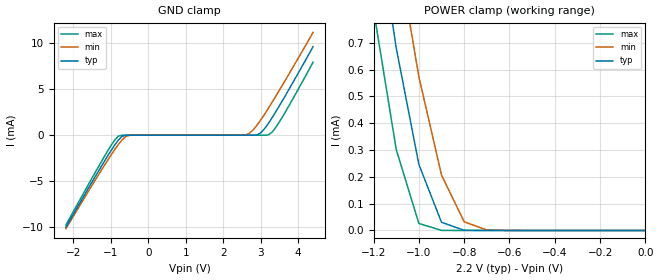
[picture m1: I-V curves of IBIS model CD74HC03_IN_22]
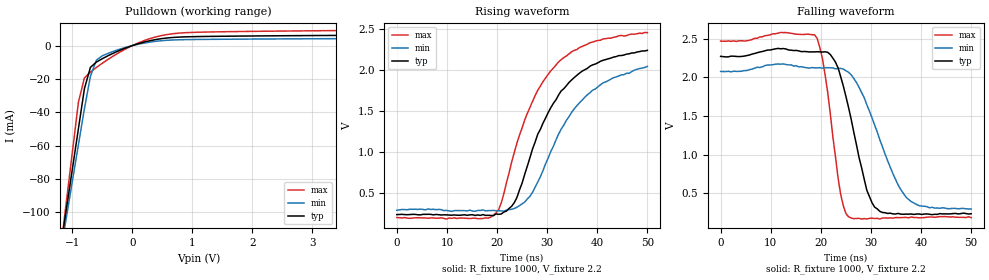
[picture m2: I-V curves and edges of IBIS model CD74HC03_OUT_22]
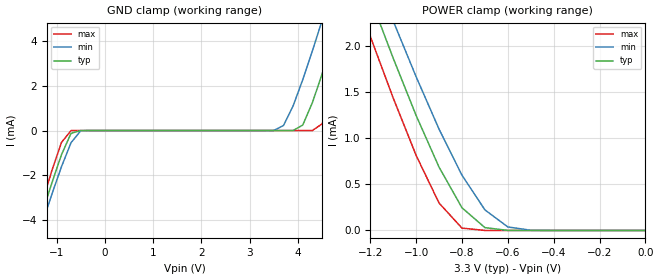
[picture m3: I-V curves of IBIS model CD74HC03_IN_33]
|   TEXAS INSTRUMENTS INCORPORATED
|   Standard Linear and Logic
|   IBIS Model of CD74HC03
|   HIGH SPEED CMOS LOGIC
|   QUAD 2-INPUT NAND GATE WITH OPEN DRAIN
|   DIP 14-pin package(N=E)
|   SOL 14-pin package(D=M)
[IBIS Ver]   3.2
[Comment Char] |_char
[File Name]   cd74hc03.ibs
[File Rev]   1.1 | x_die
[Date]   09/26/02
[Source]   File originated at Texas Instruments, Inc
[Notes]   The following is a sample IBIS file for the CD74HC03.
   - All test data contained in this file are derived from
   actual measurement.
   - The measurement used M package.
   - We have data across voltage and temperature, but not across
   process.
   - End point warnings due to AC and DC mismatch.
   - File created by Nobuhisa Ohtsubo, TIJ SLL Product Engineering.
|*   Property of Texas Instruments Incorporated.  Unauthorized
|*   reproduction and/or distribution is strictly prohibited.
|*   This product is protected under copyright law.
|*   Created 1998, (C) Copyright 1998, Texas Instruments Inc.,
|*   All Rights Reserved
|*   UNLESS THERE IS A SIGNED, WRITTEN AGREEMENT TO THE
|*   CONTRARY, TEXAS INSTRUMENTS ("TI") IS PROVIDING THE SPICE
|*   MODELS "AS IS" AND WITHOUT ANY WARRANTY, EXPRESSED OR
|*   IMPLIED.  TI assumes no liability for:
|*   1) the accuracy of the IBIS models provided to your
|*   company;
|*   2) the proper functioning of these IBIS models in your
|*   design or for any resulting applications; or
|*   3) infringement of patents, copyrights or intellectual
|*   property rights resulting from your use of these
|*   IBIS models.
|*   TI provides IBIS Models as a service to our customers.
|*   You and your company shall not distribute, sell or give
|*   these models to anyone else without prior written
|*   permission from TI.
|*   TI reserves the right to make changes to our products or
|*   to discontinue any semiconductor product or service
|*   without notice, and advises our customers to obtain the
|*   latest version of relevant information to verify, before
|*   placing orders, that the information being relied on is
|*   current.
|*   Please be aware that your receipt and use of the IBIS
|*   information provided shall serve as acceptance of these
|*   terms and conditions.  If you do not accept these terms,
|*   you should return or destroy the IBIS models and any
|*   other accompanying information immediately.
|   Component CD74HC03N (DIP)
[Component]   CD74HC03N
[Manufacturer]  Texas Instruments, Inc.
[Package]
|   typ   min   max
R_pkg   0.045   0.037   0.063
L_pkg   5.407nH   3.922nH   6.942nH
C_pkg   0.389pF   0.205pF   0.604pF
[Pin]   signal_name   model_name   R_pin   L_pin   C_pin
1   1A   CD74HC03_IN   0.063   6.942nH   0.604pF
2   1B   CD74HC03_IN   0.037   6.200nH   0.406pF
3   1Y   CD74HC03_OUT   0.042   4.389nH   0.322pF
4   2A   CD74HC03_IN   0.038   3.922nH   0.205pF
5   2B   CD74HC03_IN   0.039   4.301nH   0.298pF
6   2Y   CD74HC03_OUT   0.038   5.329nH   0.356pF
7   GND   GND   0.053   6.510nH   0.544pF
8   3Y   CD74HC03_OUT   0.053   6.437nH   0.539pF
9   3A   CD74HC03_IN   0.039   5.352nH   0.347pF
10   3B   CD74HC03_IN   0.042   4.473nH   0.297pF
11   4Y   CD74HC03_OUT   0.044   4.326nH   0.225pF
12   4A   CD74HC03_IN   0.042   4.295nH   0.280pF
13   4B   CD74HC03_IN   0.042   6.318nH   0.418pF
14   VCC   POWER   0.061   6.900nH   0.603pF
|   Component CD74HC03D (SOL)
[Component]   CD74HC03D
[Manufacturer]  Texas Instruments, Inc.
[Package]
|   typ   min   max
R_pkg   0.031   0.028   0.034
L_pkg   3.109nH   2.462nH   3.889nH
C_pkg   0.473pF   0.363pF   0.628pF
[Pin]   signal_name   model_name   R_pin   L_pin   C_pin
1   1A   CD74HC03_IN   0.033   3.854nH   0.622pF
2   1B   CD74HC03_IN   0.032   3.188nH   0.473pF
3   1Y   CD74HC03_OUT   0.028   2.462nH   0.377pF
4   2A   CD74HC03_IN   0.031   2.596nH   0.363pF
5   2B   CD74HC03_IN   0.028   2.521nH   0.372pF
6   2Y   CD74HC03_OUT   0.034   3.250nH   0.476pF
7   GND   GND   0.034   3.889nH   0.628pF
8   3Y   CD74HC03_OUT   0.034   3.889nH   0.628pF
9   3A   CD74HC03_IN   0.034   3.250nH   0.476pF
10   3B   CD74HC03_IN   0.028   2.521nH   0.372pF
11   4Y   CD74HC03_OUT   0.031   2.596nH   0.364pF
12   4A   CD74HC03_IN   0.028   2.462nH   0.377pF
13   4B   CD74HC03_IN   0.032   3.188nH   0.473pF
14   VCC   POWER   0.033   3.854nH   0.622pF
[Model Selector]   CD74HC03_IN
CD74HC03_IN_22   2.2-V Vcc Input Model
CD74HC03_IN_33   3.3-V Vcc Input Model
CD74HC03_IN_50   5.0-V Vcc Input Model
[Model Selector]   CD74HC03_OUT
CD74HC03_OUT_22   2.2-V Vcc Output Model
CD74HC03_OUT_33   3.3-V Vcc Output Model
CD74HC03_OUT_50   5.0-V Vcc Output Model
| Models and submodels in the file (6): CD74HC03_IN_22 (Input), CD74HC03_OUT_22 (Open_drain), CD74HC03_IN_33 (Input), CD74HC03_OUT_33 (Open_drain), CD74HC03_IN_50 (Input), CD74HC03_OUT_50 (Open_drain)
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|   CD74HC03 Input_IN_22
[Model]   CD74HC03_IN_22
Model_type  Input
Polarity   Inverting
Vinl = 0.5V
Vinh = 1.5V
| variable   typ   min   max
C_comp   1.526pf   1.112pf   1.907pf
[Temperature Range]   25   85   -40
[Voltage range]   2.2   2.0   2.4
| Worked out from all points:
|   GND clamp passes 1 mA (typ) near -0.88 V on its own axis
|   POWER clamp passes 1 mA (typ) near -1.16 V on its own axis
[GND Clamp]
|   Voltage   I(typ)   I(min)   I(max)
-2.2V     -10mA      -10.15mA   -9.763mA
-1.2V     -3.018mA   -3.461mA   -2.505mA
-800mV    -535.8uA   -1.021mA   -101.7uA
-700mV    -123.7uA   -510.5uA   -1.628uA
-500mV    -87.42nA   -10.24uA   17.54nA
2.5V      19.88nA    1.824uA    18.29nA
2.7V      37.79nA    206.5uA    18.36nA
3V        246.4uA    1.639mA    20.77nA
3.2V      1.24mA     2.879mA    26.21uA
3.3V      1.864mA    3.538mA    302.2uA
3.6V      3.875mA    5.559mA    2.109mA
4.4V      9.621mA    11.17mA    7.932mA
[POWER Clamp]
|   Voltage   I(typ)   I(min)   I(max)
-2.2V     8.159mA    8.344mA    7.932mA
-1.2V     1.24mA     1.639mA    823.7uA
-1.1V     681.2uA    1.071mA    302.2uA
-1V       246.4uA    573.5uA    26.21uA
-900mV    30.34uA    206.5uA    298.8nA
-800mV    887.3nA    32.29uA    20.77nA
-700mV    37.79nA    1.824uA    18.42nA
0V        19.77nA    18.03nA    18.13nA
|   Model CD74HC03 OUTPUT_22
[Model]   CD74HC03_OUT_22
Model_type  Open_drain
Polarity   Non-Inverting
Vref = 2.2
Rref = 1000
Cref = 50p
Vmeas = 1.1
| variable   typ   min   max
C_comp   1.930pf   1.534pf   2.323pf
[Temperature Range]   25   85   -40
[Voltage range]   2.2   2.0   2.4
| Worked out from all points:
|   slope of the pulldown table from 0 to 0.33 V, typ, clamps not added: 104 ohm
|   rising waveform, R_fixture 1000, V_fixture 2.2: 20-80 % time 9.16ns typ, 9.77ns min, 8.96ns max; typ from 0.237 V to 2.24 V
|   falling waveform, R_fixture 1000, V_fixture 2.2: 20-80 % time 4.22ns typ, 6.35ns min, 2.68ns max; typ from 2.27 V to 0.238 V
[Pulldown]
|   Voltage   I(typ)   I(min)   I(max)
-2.2V     -361.6mA   -340.7mA   -419.5mA
-1.2V     -121.8mA   -124.4mA   -122.9mA
-1.1V     -97.81mA   -102.8mA   -93.29mA
-900mV    -49.84mA   -59.53mA   -33.98mA
-800mV    -25.86mA   -37.91mA   -19.38mA
-700mV    -13.07mA   -18.42mA   -15.88mA
-600mV    -9.875mA   -8.728mA   -13.13mA
-500mV    -7.831mA   -6.105mA   -10.55mA
100mV     1.155mA    846.5uA    1.627mA
400mV     3.682mA    2.618mA    5.286mA
700mV     4.937mA    3.402mA    7.225mA
4.4V      6.306mA    4.299mA    9.265mA
[ramp]
| variable   typ   min   max
dV/dt_r   1.224E+00/8.759E-09  1.068E+00/9.062E-09  1.386E+00/8.521E-09
dV/dt_f   1.284E+00/4.146E-09  1.200E-01/7.252E-09  1.398E+00/2.603E-09
[Rising Waveform]
R_fixture = 1000
V_fixture = 2.2
V_fixture_min = 2.0
V_fixture_max = 2.4
C_fixture = 0
L_fixture = 0
|   Time   V(typ)   V(min)   V(max)
0s        237.4mV    290.7mV    201.6mV
18.75ns   227.2mV    286.4mV    207.2mV
20.83ns   244.6mV    282.6mV    378mV
23.44ns   382.7mV    312mV      994mV
27.08ns   1.036V     508.6mV    1.615V
30.73ns   1.54V      1.007V     1.988V
33.85ns   1.808V     1.386V     2.169V
38.02ns   2.018V     1.696V     2.312V
43.23ns   2.155V     1.904V     2.396V
50ns      2.237V     2.042V     2.453V
[Falling Waveform]
R_fixture = 1000
V_fixture = 2.2
V_fixture_min = 2.0
V_fixture_max = 2.4
C_fixture = 0
L_fixture = 0
|   Time   V(typ)   V(min)   V(max)
0s        2.272V     2.077V     2.469V
18.75ns   2.33V      2.124V     2.551V
20.31ns   2.328V     2.119V     2.246V
22.92ns   2.197V     2.111V     971.1mV
23.96ns   2.008V     2.116V     486.2mV
25.52ns   1.613V     2.067V     199.3mV
29.17ns   541.7mV    1.647V     170.1mV
30.73ns   323.6mV    1.384V     175.6mV
37.5ns    232.2mV    423mV      185.5mV
50ns      238.2mV    299.4mV    187.7mV
|   CD74HC03 Input_IN_33
[Model]   CD74HC03_IN_33
Model_type  Input
Polarity   Inverting
Vinl = 1.35V
Vinh = 3.15V
| variable   typ   min   max
C_comp   1.526pf   1.112pf   1.907pf
[Temperature Range]   25   85   -40
[Voltage range]   3.3   3.0   3.6
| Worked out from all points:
|   GND clamp passes 1 mA (typ) near -0.88 V on its own axis
|   POWER clamp passes 1 mA (typ) near -0.96 V on its own axis
[GND Clamp]
|   Voltage   I(typ)   I(min)   I(max)
-3.3V     -17.81mA   -17.63mA   -17.87mA
-1.5V     -5.078mA   -5.462mA   -4.636mA
-900mV    -1.088mA   -1.622mA   -537.2uA
-700mV    -123.3uA   -541.4uA   -1.421uA
3.5V      19.41nA    2.345uA    19.74nA
3.7V      19.86nA    223.2uA    19.8nA
4.1V      246uA      2.27mA     19.85nA
4.3V      1.246mA    3.557mA    278.8nA
4.5V      2.521mA    4.899mA    297.5uA
4.7V      3.879mA    6.265mA    1.436mA
5.1V      6.714mA    9.051mA    4.226mA
6.6V      17.72mA    19.7mA     15.5mA
[POWER Clamp]
|   Voltage   I(typ)   I(min)   I(max)
-3.3V     17.72mA    17.57mA    17.78mA
-1.3V     3.189mA    3.557mA    2.8mA
-1.2V     2.521mA    2.905mA    2.104mA
-1.1V     1.867mA    2.27mA     1.436mA
-1V       1.246mA    1.666mA    813.7uA
-900mV    686.5uA    1.098mA    297.5uA
-800mV    246uA      598.8uA    25.57uA
-700mV    30.98uA    223.2uA    278.8nA
-600mV    917nA      38.1uA     21.8nA
-500mV    37.7nA     2.345uA    19.85nA
0V        19.41nA    20.03nA    19.78nA
